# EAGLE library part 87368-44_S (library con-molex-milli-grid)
RECEPTACAL
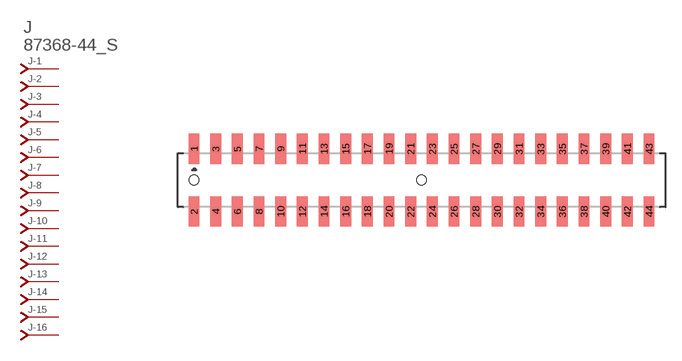
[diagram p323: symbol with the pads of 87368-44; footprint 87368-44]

Designator prefix J; gates -1=J-NV -2=J-N -3=J-N -4=J-N -5=J-N -6=J-N -7=J-N -8=J-N -9=J-N -10=J-N -11=J-N -12=J-N -13=J-N -14=J-N -15=J-N -16=J-N -17=J-N -18=J-N -19=J-N -20=J-N -21=J-N -22=J-N -23=J-N -24=J-N -25=J-N -26=J-N -27=J-N -28=J-N -29=J-N -30=J-N -31=J-N -32=J-N -33=J-N -34=J-N -35=J-N -36=J-N -37=J-N -38=J-N -39=J-N -40=J-N -41=J-N -42=J-N -43=J-N -44=J-N

## 87368-44_S  [87368-44]
1  -1:J  pas
2  -2:J  pas
3  -3:J  pas
4  -4:J  pas
5  -5:J  pas
6  -6:J  pas
7  -7:J  pas
8  -8:J  pas
9  -9:J  pas
10  -10:J  pas
11  -11:J  pas
12  -12:J  pas
13  -13:J  pas
14  -14:J  pas
15  -15:J  pas
16  -16:J  pas
17  -17:J  pas
18  -18:J  pas
19  -19:J  pas
20  -20:J  pas
21  -21:J  pas
22  -22:J  pas
23  -23:J  pas
24  -24:J  pas
25  -25:J  pas
26  -26:J  pas
27  -27:J  pas
28  -28:J  pas
29  -29:J  pas
30  -30:J  pas
31  -31:J  pas
32  -32:J  pas
33  -33:J  pas
34  -34:J  pas
35  -35:J  pas
36  -36:J  pas
37  -37:J  pas
38  -38:J  pas
39  -39:J  pas
40  -40:J  pas
41  -41:J  pas
42  -42:J  pas
43  -43:J  pas
44  -44:J  pas

## Footprint 87368-44 (pad centres in mm)
RECEPTACAL SMD Dual Row, Side Entry
smd 1 x 2.8: 1 -21,2.9; 2 -21,-2.9; 3 -19,2.9; 4 -19,-2.9; 5 -17,2.9; 6 -17,-2.9; 7 -15,2.9; 8 -15,-2.9; 9 -13,2.9; 10 -13,-2.9; 11 -11,2.9; 12 -11,-2.9; 13 -9,2.9; 14 -9,-2.9; 15 -7,2.9; 16 -7,-2.9; 17 -5,2.9; 18 -5,-2.9; 19 -3,2.9; 20 -3,-2.9; 21 -1,2.9; 22 -1,-2.9; 23 1,2.9; 24 1,-2.9; 25 3,2.9; 26 3,-2.9; 27 5,2.9; 28 5,-2.9; 29 7,2.9; 30 7,-2.9; 31 9,2.9; 32 9,-2.9; 33 11,2.9; 34 11,-2.9; 35 13,2.9; 36 13,-2.9; 37 15,2.9; 38 15,-2.9; 39 17,2.9; 40 17,-2.9; 41 19,2.9; 42 19,-2.9; 43 21,2.9; 44 21,-2.9
hole 0.914 at -21,0
hole 0.914 at 0,0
